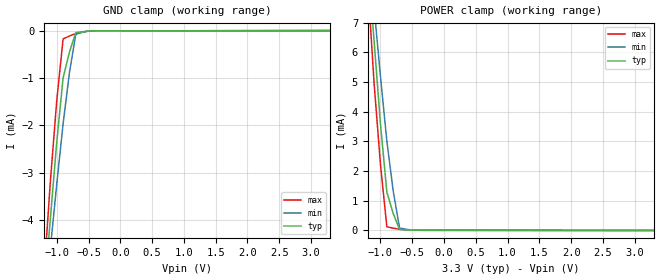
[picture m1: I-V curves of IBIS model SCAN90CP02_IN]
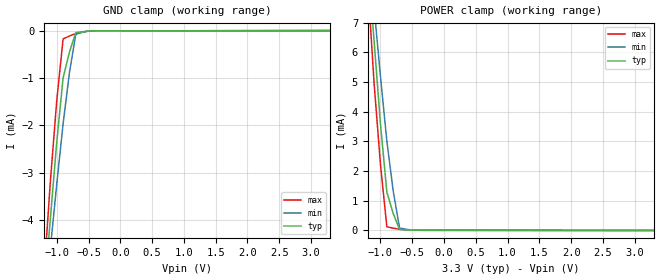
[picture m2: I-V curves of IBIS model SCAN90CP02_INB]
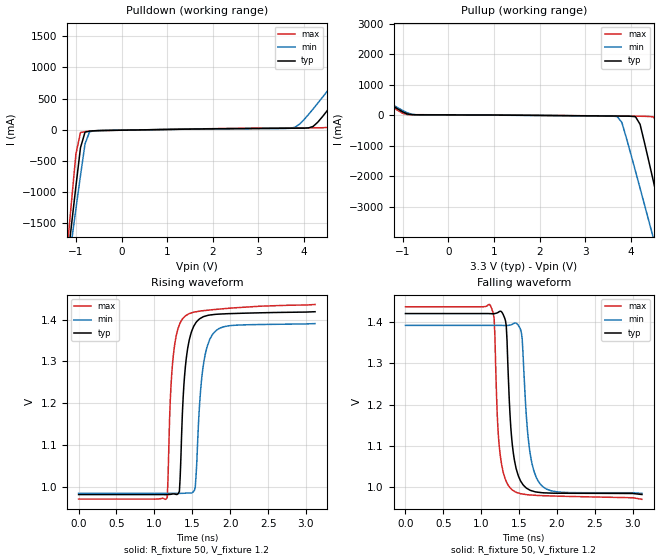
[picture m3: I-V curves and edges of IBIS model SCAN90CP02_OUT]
|   National Semiconductor Corporation
|   IBIS Model
|   of
|   SCAN90CP02
|   1.5Gbps 2x2 LVDS Crosspoint Switch
|   with Pre-emphasis and IEEE1149.6
|   28 pin LLP package
[IBIS Ver]   3.2
[Comment Char]   |_char
[File name]   scan90cp02.ibs
[File Rev]   2.0
[Date]   08/14/07
[Source]
SpectreS simulation, Bench data
IEEE1149.1 cells created from SCAN928028
[Notes]
R1.0   10/25/03   Created. -I.D.
R2.0   08/14/07   Updated SCAN90CP02_OUT model, added SCAN90CP02_OUTB &
   SCAN90CP02_INB models, fixed min/max columns. -J.T.B.
[Disclaimer]
(C) Copyright National Semiconductor Corporation 2002
   All rights reserved
   National Semiconductor Corporation hereby grants
the user of this IBIS model a non-exclusive, nontransferable
license to use this IBIS model under the following terms.
Before using this IBIS model, the user should read this
license.  If the user does not accept these terms,  the
IBIS model should be returned to National within 30 days.
   The user is granted this license only to use the
IBIS model and is not granted rights to sell, load, rent,
lease or license the IBIS model in whole or in part, or in
modified form to anyone other than user. User may modify
the IBIS model to suit its specific applications but rights
to derivative works and such modifications shall belong to
National.
   This IBIS model is provided on an "AS IS" basis and
National makes absolutely no warranty with respect to the
information contained herein.NATIONAL DISCLAIMS AND CUSTOMER
WAIVES ALL WARRANTIES, EXPRESS OR IMPLIED, INCLUDING
WARRANTIES OF MERCHANTABILITY OR FITNESS FOR A PARTICULAR
PURPOSE. The entire risk as to quality and performance is
with the Customer. ACCORDINGLY, IN NO EVENT SHALL THE
COMPANY BE LIABLE FOR ANY DAMAGES, WHETHER IN CONTRACT OR
TORT,INCLUDING ANY LOST PROFITS OR OTHER INCIDENTAL,
CONSEQUENTIAL, EXEMPLARY, OR PUNITIVE DAMAGES ARISING OUT
OF THE USE OR APPLICATION OF THE IBIS model provided in
this package.Further, National reserves the right to make
changes without notice to any product herein to improve
reliability, function, or design. National does not convey
any license under patent rights or any other intellectual
property rights, including those of third parties.
   National is not obligated to provide maintenance or support
for the licensed IBIS model.
Contact National at ATTN:ENHANCED SOLUTIONS/IBIS MODELS.
5 Foden Road, M/S 01-50, South Porltand, ME 04106
[Copyright]
(c) Copyright 2002 National Semiconductor Corp.
[Component]   SCAN90CP02
Si_location Pin
Timing_location Pin
[Manufacturer]   National Semiconductor Corp.
[Package]
|   TYP   MIN   MAX
R_pkg   100.0m   100.0m   100.0m
L_pkg   1nH   1nH   1nH
C_pkg   0.2pF   0.2pF   0.2pF
[Pin]   signal_name   model_name   R_pin   L_pin   C_pin
1   PEM11   SCAN90CP02_SEL
2   PEM10   SCAN90CP02_SEL
3   PEM01   SCAN90CP02_SEL
4   PEM00   SCAN90CP02_SEL
5   SEL1   SCAN90CP02_SEL
6   SEL0   SCAN90CP02_SEL
7   EN0b   SCAN90CP02_SEL
8   NC   NC
9   IN0+   SCAN90CP02_IN
10   IN0-   SCAN90CP02_INB
11   VDDA   POWER
12   IN1+   SCAN90CP02_IN
13   IN1-   SCAN90CP02_INB
14   VDD2   POWER
15   EN1b   SCAN90CP02_SEL
16   VDD1   POWER
17   TCK   SCAN90CP02_SEL
18   TMS   SCAN90CP02_SEL
19   TDI   SCAN90CP02_SEL
20   TDO   SCAN90CP02_JTAGOUT
21   TRSTb   SCAN90CP02_SEL
22   VDD2   POWER
23   OUT1-   SCAN90CP02_OUTB
24   OUT1+   SCAN90CP02_OUT
25   VDDA   POWER
26   OUT0-   SCAN90CP02_OUTB
27   OUT0+   SCAN90CP02_OUT
28   NC   NC
[Diff Pin] inv_pin   vdiff   tdelay_typ   tdelay_min   tdelay_max
| The '+' pin is Diff_pin and the '-' pin is the inv_pin
| Receiver Vth = +/-100mV
9   10   0.05   0   0   0
12   13   0.05   0   0   0
24   23   0.00   0   0   0
27   26   0.00   0   0   0
| Models and submodels in the file (6): SCAN90CP02_IN (Input), SCAN90CP02_INB (Input), SCAN90CP02_OUT (Output), SCAN90CP02_OUTB (Output), SCAN90CP02_JTAGOUT (Output), SCAN90CP02_SEL (Input)
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[Model]   SCAN90CP02_IN
Model_type Input
Polarity Non-Inverting
Vinh=0.05
Vinl=-0.05
C_comp   5pF   5pF   5pF
[Temperature Range] 25   85   -40
[Voltage Range]   3.3   3.0   3.6
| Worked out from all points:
|   GND clamp passes 1 mA (typ) near -0.90 V on its own axis
|   POWER clamp passes 1 mA (typ) near -0.86 V on its own axis
[GND Clamp]
|V(groundclamp)   I(typ)   I(min)   I(max)
-3.3V     -39.4mA    -34.1mA    -48.4mA
-1.2V     -5.59mA    -5.94mA    -5.16mA
-1.1V     -3.97mA    -4.6mA     -3.18mA
-1V       -2.36mA    -3.25mA    -1.48mA
-900mV    -999uA     -1.97mA    -174uA
-800mV    -452uA     -888uA     -113uA
-700mV    -42uA      -77.3uA    -60.2uA
-500mV    -8.18uA    -6.08uA    -10.7uA
3.3V      1.65uA     1.37uA     2.08uA
[POWER Clamp]
|Vtable   I(typ)   I(min)   I(max)
-3.3V     67.6mA     58.5mA     82.8mA
-1.2V     9.15mA     9.82mA     8.31mA
-1.1V     6.36mA     7.5mA      4.94mA
-1V       3.58mA     5.18mA     2.21mA
-900mV    1.29mA     3.01mA     121uA
-800mV    569uA      1.33mA     75.2uA
-700mV    31.3uA     82.2uA     36.8uA
-500mV    6.39uA     5.42uA     7.01uA
3.3V      -3.3uA     -2.73uA    -4.15uA
[Model]   SCAN90CP02_INB
Model_type Input
Polarity Inverting
Vinh=0.05
Vinl=-0.05
C_comp   5pF   5pF   5pF
[Temperature Range] 25   85   -40
[Voltage Range]   3.3   3.0   3.6
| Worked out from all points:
|   GND clamp passes 1 mA (typ) near -0.90 V on its own axis
|   POWER clamp passes 1 mA (typ) near -0.86 V on its own axis
[GND Clamp]
|V(groundclamp)   I(typ)   I(min)   I(max)
-3.3V     -39.4mA    -34.1mA    -48.4mA
-1.2V     -5.59mA    -5.94mA    -5.16mA
-1.1V     -3.97mA    -4.6mA     -3.18mA
-1V       -2.36mA    -3.25mA    -1.48mA
-900mV    -999uA     -1.97mA    -174uA
-800mV    -452uA     -888uA     -113uA
-700mV    -42uA      -77.3uA    -60.2uA
-500mV    -8.18uA    -6.08uA    -10.7uA
3.3V      1.65uA     1.37uA     2.08uA
[POWER Clamp]
|Vtable   I(typ)   I(min)   I(max)
-3.3V     67.6mA     58.5mA     82.8mA
-1.2V     9.15mA     9.82mA     8.31mA
-1.1V     6.36mA     7.5mA      4.94mA
-1V       3.58mA     5.18mA     2.21mA
-900mV    1.29mA     3.01mA     121uA
-800mV    569uA      1.33mA     75.2uA
-700mV    31.3uA     82.2uA     36.8uA
-500mV    6.39uA     5.42uA     7.01uA
3.3V      -3.3uA     -2.73uA    -4.15uA
[Model]   SCAN90CP02_OUT
Model_type Output
Polarity Non-Inverting
Vref=1.2
Vmeas=1.2
Rref=50   | 100 Ohms Across Outputs OUT+ and OUT-
Cref=1p
C_comp   8pF   8pF   8pF
[Temperature Range] 25   85   -40
[Voltage Range]   3.3   3.0   3.6
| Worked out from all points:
|   slope of the pulldown table from 0 to 0.495 V, typ, clamps not added: 84.1 ohm
|   slope of the pullup table from 0 to 0.495 V, typ, clamps not added: 210 ohm
|   falling waveform, R_fixture 50, V_fixture 1.2: 20-80 % time 89.6ps typ, 105ps min, 77.8ps max; typ from 1.42 V to 0.983 V
|   rising waveform, R_fixture 50, V_fixture 1.2: 20-80 % time 89.8ps typ, 101ps min, 83.9ps max; typ from 0.981 V to 1.42 V
[Pulldown]
|V(pulldown)   I(typ)   I(min)   I(max)
-3.6V     -17.92A    -15.75A    -21.54A
-1.2V     -2.195A    -2.367A    -1.985A
-1.1V     -1.548A    -1.817A    -1.18A
-1V       -908.9mA   -1.271A    -391.3mA
-900mV    -289.9mA   -736mA     -45.84mA
-700mV    -22.24mA   -32.94mA   -22.09mA
3.7V      24.24mA    23.61mA    28.16mA
4.5V      299.2mA    610.9mA    36.3mA
5.6V      1.408A     1.668A     1.121A
5.8V      1.614A     1.863A     1.342A
6.1V      1.925A     2.156A     1.675A
7.2V      3.072A     3.237A     2.903A
[Pullup]
|V(pullup)   I(typ)   I(min)   I(max)
-3.6V     2.74A      2.632A     2.88A
-900mV    43.34mA    80.56mA    22.72mA
3.7V      -26.74mA   -42.08mA   -25.25mA
3.8V      -28.09mA   -232.2mA   -26.59mA
4.1V      -47.53mA   -1.832A    -30.63mA
4.2V      -296.4mA   -2.387A    -32.38mA
4.5V      -2.212A    -4.064A    -54.8mA
4.6V      -2.868A    -4.625A    -397.6mA
4.8V      -4.186A    -5.747A    -1.996A
5V        -5.506A    -6.87A     -3.632A
5.1V      -6.167A    -7.431A    -4.453A
7.2V      -19.97A    -19.17A    -21.64A
[Ramp]
|   typ   min   max
dV/dt_r   320mV/.145ns   310mV/.160ns   330mV/0.120ns
dV/dt_f   320mv/.120ns   310mv/.130ns   330mv/0.100ns
R_load=50
[Falling Waveform]
R_fixture=50
V_fixture=1.2
V_fixture_min=1.18814
V_fixture_max=1.20375
0s        1.421V     1.392V     1.437V
1.12ns    1.421V     1.392V     1.44V
1.17ns    1.421V     1.392V     1.408V
1.23ns    1.425V     1.392V     1.116V
1.32ns    1.403V     1.392V     1.019V
1.41ns    1.103V     1.395V     993.8mV
1.53ns    1.012V     1.374V     984.5mV
1.63ns    994.8mV    1.102V     982mV
1.78ns    987.8mV    1.008V     980.3mV
3.12ns    982.9mV    985.7mV    971.3mV
[Rising Waveform]
R_fixture=50
V_fixture=1.2
V_fixture_min=1.2
V_fixture_max=1.2
0s        981.3mV    984.2mV    970.5mV
1.17ns    981.3mV    984.2mV    974.8mV
1.23ns    982.5mV    984.2mV    1.273V
1.33ns    989.2mV    984.1mV    1.388V
1.37ns    1.178V     984.3mV    1.402V
1.41ns    1.289V     984.8mV    1.409V
1.54ns    1.391V     1.001V     1.419V
1.63ns    1.406V     1.269V     1.421V
1.78ns    1.412V     1.368V     1.424V
3.12ns    1.419V     1.391V     1.436V
